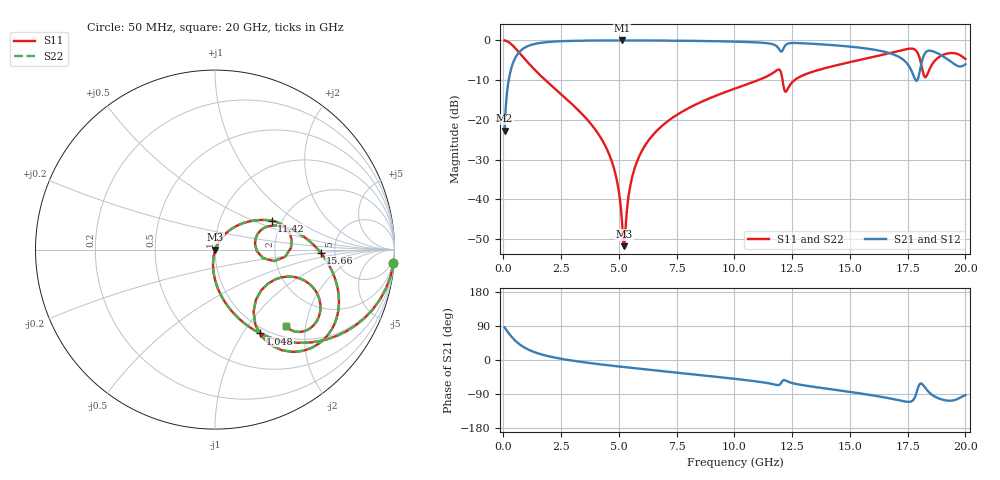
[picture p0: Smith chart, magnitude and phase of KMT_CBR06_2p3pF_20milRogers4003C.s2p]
! Data measured by Modelithics Inc. support@modelithics.com 813-866-6335
! KEMET CBR0603 2.3pF, Pad Width= 0.851mm, Pad Length= 0.64mm, Pad Gap= 0.62mm, 20mil Rogers 4003C substrate Data, January 2022
# hz S ma R 50
! 2 Port Network Data from SP1.SP block
! freq  magS11  angS11  magS21  angS21  magS12  angS12  magS22  angS22
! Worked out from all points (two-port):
!   401 points, 50 MHz to 20 GHz, reference 50 ohm
!   highest |S21| = -0.02 dB at 5.137 GHz (marker M1); lowest = -22.7 dB at 50 MHz (marker M2)
!   |S21| within 3 dB of the highest: 672.9 MHz to 16.6 GHz (15.93 GHz wide, 184 % of centre); 18.28 GHz to 18.71 GHz (427.6 MHz wide, 2.31 % of centre)
!   lowest |S11| = -51.8 dB at 5.237 GHz (marker M3), VSWR 1.01, Z = 50.3 + j0.0184 ohm
!   |S11| at or under -10 dB: 1.817 GHz to 11.03 GHz (9.212 GHz wide, 143 % of centre); 12.08 GHz to 12.6 GHz (520.9 MHz wide, 4.22 % of centre)
!   |S22| runs from -51.8 to 0.0 dB; largest |S21 - S12| = 0
!   S11 on the Smith chart (normalised r, x): 50 MHz: 1, -26; 1.048 GHz: 0.93, -1.20; 11.42 GHz: 1.77, +0.65; 15.66 GHz: 3.85, -0.19; 20 GHz: 1.21, -1.57
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5e7  0.9973 -4.4  0.07302 85.6  0.07302 85.6  0.9973 -4.4
3.99125e8  0.8617 -31.8  0.5063 58.1  0.5063 58.1  0.8617 -31.8
1.0475e9  0.5312 -61.5  0.8459 28.3  0.8459 28.3  0.5312 -61.5
3.391625e9  0.1196 -94.3  0.9907 -5.3  0.9907 -5.3  0.1196 -94.3
4.6385e9  0.03312 -100.8  0.997 -14.7  0.997 -14.7  0.03312 -100.8
4.93775e9  0.01581 -98.3  0.9974 -16.7  0.9974 -16.7  0.01581 -98.3
5.13725e9  0.005054 -80.2  0.9974 -18.1  0.9974 -18.1  0.005054 -80.2
5.237e9  0.002583 4.1  0.9974 -18.7  0.9974 -18.7  0.002583 4.1
5.73575e9  0.02756 62.8  0.9969 -22.0  0.9969 -22.0  0.02756 62.8
6.73325e9  0.07758 59.6  0.994 -28.4  0.994 -28.4  0.07758 59.6
1.0025e10  0.248 39.3  0.9641 -49.7  0.9641 -49.7  0.248 39.3
1.14215e10  0.3543 27.0  0.9211 -60.8  0.9211 -60.8  0.3543 27.0
1.192025e10  0.4309 7.4  0.7879 -66.1  0.7879 -66.1  0.4309 7.4
1.226938e10  0.2343 15.1  0.8977 -55.7  0.8977 -55.7  0.2343 15.1
1.336662e10  0.4013 18.4  0.906 -70.2  0.906 -70.2  0.4013 18.4
1.566088e10  0.5884 -1.6  0.7937 -90.2  0.7937 -90.2  0.5884 -1.6
1.670825e10  0.6892 -13.8  0.6922 -101.1  0.6922 -101.1  0.6892 -13.8
1.785538e10  0.7479 -48.9  0.3122 -91.9  0.3122 -91.9  0.7479 -48.9
1.815462e10  0.4078 -58.2  0.5933 -64.9  0.5933 -64.9  0.4078 -58.2
1.845388e10  0.4367 -20.1  0.7426 -86.8  0.7426 -86.8  0.4367 -20.1
1.895262e10  0.6404 -25.1  0.6504 -103.6  0.6504 -103.6  0.6404 -25.1
2e10  0.5834 -47.0  0.5007 -92.8  0.5007 -92.8  0.5834 -47.0
